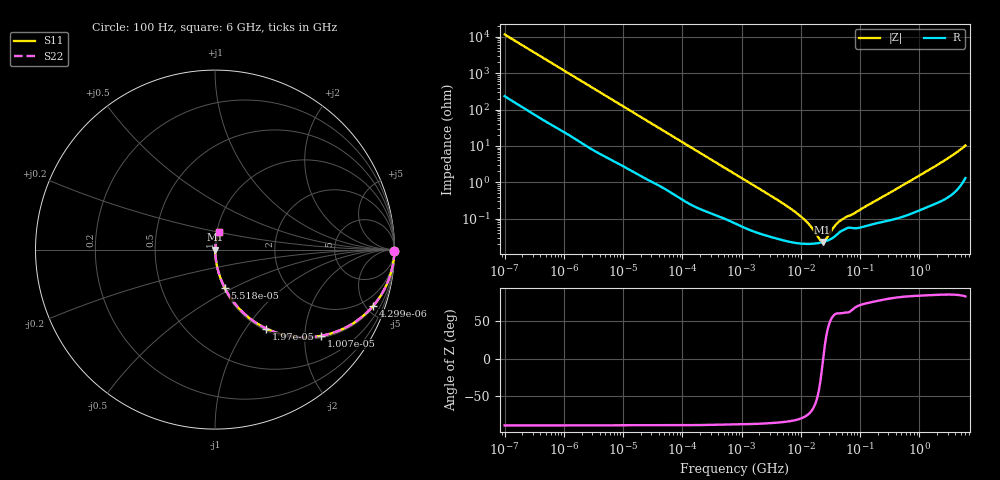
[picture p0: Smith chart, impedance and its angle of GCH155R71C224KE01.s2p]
!Murata Part Number: GCH155R71C224KE01
!These Parameters are Measured in Series Mode Connection
!Data Generated on Jun 19, 2026
!  o--ll--o
!Port1  Port2
!  o------o
!Operation Temp=25[degC], DC Bias Voltage=0[V]
!Freq. Start=100[Hz] Stop=6[GHz] 401[Steps]
# Hz S RI R 50
!Freq.(Hz) S11(Real) S11(Imag) S21(Real) S21(Imag) S12(Real) S12(Imag) S22(Real) S22(Imag)
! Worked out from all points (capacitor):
!   401 points, 100 Hz to 6 GHz, reference 50 ohm
!   read as one part in series: C = 138 nF near 109 Hz
!   lowest |Z| = 23 mohm at 23.28 MHz (marker M1)
!   series resonance near 23.86 MHz, so ESL is about 320 pH
!   S11 on the Smith chart (normalised r, x): 100 Hz: open; 4.299 kHz: 1.12, -5.60; 10.07 kHz: 1.06, -2.42; 19.7 kHz: 1.03, -1.25; 55.18 kHz: 1.01, -0.45; 6 GHz: 1.03, +0.20
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100  0.9997 -0.00869  0.000252 0.00869  0.000252 0.00869  0.9997 -0.00869
600  0.9964 -0.0508  0.0036 0.0508  0.0036 0.0508  0.9964 -0.0508
2008  0.9694 -0.1624  0.0306 0.1624  0.0306 0.1624  0.9694 -0.1624
4299  0.8821 -0.3124  0.1179 0.3124  0.1179 0.3124  0.8821 -0.3124
6433  0.775 -0.4069  0.225 0.4069  0.225 0.4069  0.775 -0.4069
10066  0.5925 -0.4801  0.4075 0.4801  0.4075 0.4801  0.5925 -0.4801
19704  0.2853 -0.4397  0.7147 0.4397  0.7147 0.4397  0.2853 -0.4397
40335  0.0931 -0.2776  0.9069 0.2776  0.9069 0.2776  0.0931 -0.2776
55182  0.0542 -0.2133  0.9458 0.2133  0.9458 0.2133  0.0542 -0.2133
161617  0.00827 -0.0779  0.9917 0.0779  0.9917 0.0779  0.00827 -0.0779
774597  0.00103 -0.0169  0.999 0.0169  0.999 0.0169  0.00103 -0.0169
6644369  0.000234 -0.00191  0.9998 0.00191  0.9998 0.00191  0.000234 -0.00191
1.087309e7  0.000207 -0.00101  0.9998 0.00101  0.9998 0.00101  0.000207 -0.00101
1.555665e7  0.000206 -0.000514  0.9998 0.000514  0.9998 0.000514  0.000206 -0.000514
2.035112e7  0.000217 -0.000186  0.9998 0.000186  0.9998 0.000186  0.000217 -0.000186
2.327686e7  0.000228 -2.87e-05  0.9998 2.87e-05  0.9998 2.87e-05  0.000228 -2.87e-05
2.545746e7  0.000237 7.6e-05  0.9998 -7.6e-05  0.9998 -7.6e-05  0.000237 7.6e-05
3.64232e7  0.000317 0.000506  0.9997 -0.000506  0.9997 -0.000506  0.000317 0.000506
4.764863e7  0.000456 0.000793  0.9995 -0.000793  0.9995 -0.000793  0.000456 0.000793
3.124326e8  0.000926 0.005  0.9991 -0.005  0.9991 -0.005  0.000926 0.005
2.240541e9  0.00404 0.0331  0.996 -0.0331  0.996 -0.0331  0.00404 0.0331
6e9  0.0228 0.0983  0.9772 -0.0983  0.9772 -0.0983  0.0228 0.0983
